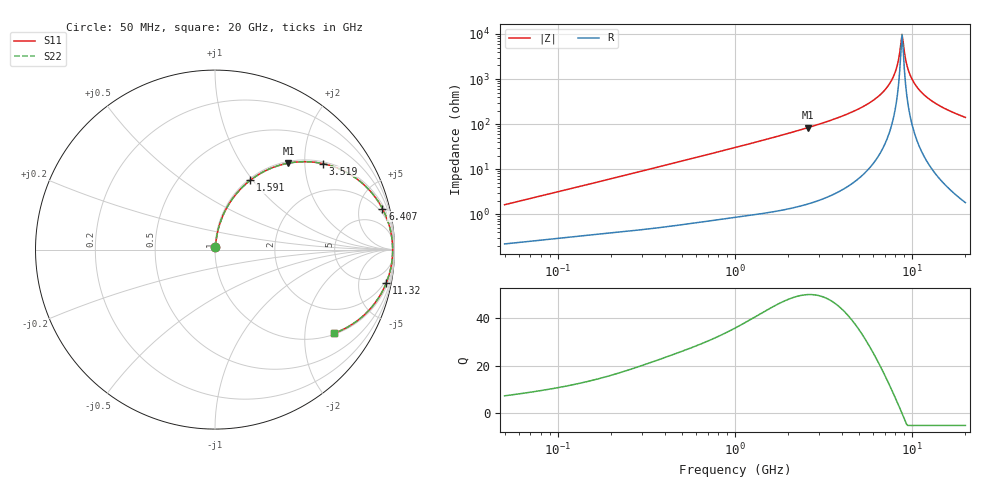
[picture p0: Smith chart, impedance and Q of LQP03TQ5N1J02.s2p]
!Murata Part Number: LQP03TQ5N1J02
!These Parameters are Measured in Series Mode Connection
!  o--[Z]--o
!Port1  Port2
!  o-------o
!Freq. Start=50[MHz] Stop=20[GHz], 401[Steps]
# Hz S RI R 50
!Freq.(Hz) S11(Real) S11(Imag) S21(Real) S21(Imag) S12(Real) S12(Imag) S22(Real) S22(Imag)
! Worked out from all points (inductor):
!   401 points, 50 MHz to 20 GHz, reference 50 ohm
!   read as one part in series: L = 5.06 nH near 51.52 MHz
!   highest Q = 49.6 at 2.569 GHz (marker M1), where L = 5.13 nH
!   self-resonance near 8.775 GHz
!   S11 on the Smith chart (normalised r, x): 50 MHz: 1.00, +0.03; 1.591 GHz: 1.02, +0.97; 3.519 GHz: 1.05, +2.47; 6.407 GHz: 1.37, +8.05; 11.32 GHz: 1, -10; 20 GHz: 1.04, -2.81
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5e7  0.00243 0.016  0.9976 -0.016  0.9976 -0.016  0.00243 0.016
1.364002e8  0.00505 0.0418  0.9949 -0.0418  0.9949 -0.0418  0.00505 0.0418
3.721004e8  0.0173 0.11  0.9827 -0.11  0.9827 -0.11  0.0173 0.11
1e9  0.0895 0.2718  0.9105 -0.2718  0.9105 -0.2718  0.0895 0.2718
1.590961e9  0.1968 0.3864  0.8032 -0.3864  0.8032 -0.3864  0.1968 0.3864
2.569357e9  0.409 0.4817  0.591 -0.4817  0.591 -0.4817  0.409 0.4817
2.728004e9  0.4433 0.4868  0.5567 -0.4868  0.5567 -0.4868  0.4433 0.4868
3.519108e9  0.602 0.4789  0.398 -0.4789  0.398 -0.4789  0.602 0.4789
4.966507e9  0.8153 0.3742  0.1847 -0.3742  0.1847 -0.3742  0.8153 0.3742
6.406762e9  0.9327 0.2286  0.0673 -0.2286  0.0673 -0.2286  0.9327 0.2286
7.442007e9  0.9736 0.1239  0.0264 -0.1239  0.0264 -0.1239  0.9736 0.1239
8.020766e9  0.9848 0.0684  0.0152 -0.0684  0.0152 -0.0684  0.9848 0.0684
8.264682e9  0.9876 0.0459  0.0124 -0.0459  0.0124 -0.0459  0.9876 0.0459
8.644534e9  0.9897 0.0119  0.0103 -0.0119  0.0103 -0.0119  0.9897 0.0119
8.774992e9  0.9899 0.00059  0.0101 -0.00059  0.0101 -0.00059  0.9899 0.00059
9.041845e9  0.9895 -0.0221  0.0105 0.0221  0.0105 0.0221  0.9895 -0.0221
9.316812e9  0.988 -0.0448  0.012 0.0448  0.012 0.0448  0.988 -0.0448
9.745021e9  0.9839 -0.0786  0.0161 0.0786  0.0161 0.0786  0.9839 -0.0786
1.034674e10  0.9747 -0.123  0.0253 0.123  0.0253 0.123  0.9747 -0.123
1.131968e10  0.9536 -0.1874  0.0464 0.1874  0.0464 0.1874  0.9536 -0.1874
1.438523e10  0.8577 -0.3377  0.1423 0.3377  0.1423 0.3377  0.8577 -0.3377
2e10  0.6622 -0.4666  0.3378 0.4666  0.3378 0.4666  0.6622 -0.4666
